(* Logix 5000 AddOnInstructionDefinition export Banner_TL70PS_PD_v6; software revision 33.00 *)

TYPE Banner_TL70PS_Adv_PD_Seg_v6 :   // Advanced process data set for a TL70 Pro Select Segment.
STRUCT
   Animation : SINT;   // 0 = Off, 1 = Steady, 2 = Flash, 3 = Two Color Flash, 4 = Half/Half, 5 = Half/Half Rotate, 6 = Chase, 7 = Intesnity Sweep
   Speed : SINT;   // 0 = Medium, 1 = Slow, 2 = Fast, 3 = Custom
   Pattern : SINT;   // 0 = Normal, 1 = Strobe, 2 = Three Pulse, 3 = SOS, 4 = Random
   Color_1 : SINT;   // 0=Green, 1=Red, 2=Orange, 3=Amber, 4=Yellow, 5=Lime Green, 6=Spring Green, 7=Cyan, 8=Sky Blue, 9=Blue, 10=Violet, 11=Magenta, 12=Rose, 13 = White
   Color_1_Intensity : SINT;   // 0=High, 1=Medium, 2=Low, 3 = Off, 4 = Custom
   Color_2 : SINT;   // 0=Green, 1=Red, 2=Orange, 3=Amber, 4=Yellow, 5=Lime Green, 6=Spring Green, 7=Cyan, 8=Sky Blue, 9=Blue, 10=Violet, 11=Magenta, 12=Rose, 13 = White
   Color_2_Instensity : SINT;   // 0=High, 1=Medium, 2=Low, 3 = Off, 4 = Custom
END_STRUCT
END_TYPE

TYPE Banner_TL70PS_Adv_PDO_v6 :   // Advanced process data set for a TL70 Pro Select IO-Link unit.
STRUCT
   Segment_1 : Banner_TL70PS_Adv_PD_Seg_v6;   // Advanced process data set for a TL70 Segment.
   Segment_2 : Banner_TL70PS_Adv_PD_Seg_v6;   // Advanced process data set for a TL70 Segment.
   Segment_3 : Banner_TL70PS_Adv_PD_Seg_v6;   // Advanced process data set for a TL70 Segment.
   Segment_4 : Banner_TL70PS_Adv_PD_Seg_v6;   // Advanced process data set for a TL70 Segment.
   Segment_5 : Banner_TL70PS_Adv_PD_Seg_v6;   // Advanced process data set for a TL70 Segment.
   Audible_State : SINT;   // 0 = Off, 1 = On
   Audible_Type : SINT;   // 0=Freq, 1=Sync, 2=Off
   Audible_Volume : SINT;   // 0=High, 1=Medium, 2=Low, 3=Off
   Audible_Tone_1 : SINT;   // 0=Freq 3, 1=Freq 2, 2=Freq 1, 3=Off
   Audible_Tone_2 : SINT;   // 0=Freq 3, 1=Freq 2, 2=Freq 1, 3=Off
END_STRUCT
END_TYPE

TYPE Banner_TL70PS_Out_Level_v6 :
STRUCT
   Process_Level : INT;
   Audible_State : SINT;   // 0=Off, 1=On
END_STRUCT
END_TYPE

TYPE Banner_TL70PS_PDO_v6 :   // Process data for a Banner TL70 Pro Select unit. This includes four process data types.
STRUCT
   Segment_PD : Banner_TL70PS_Segment_PD_v6;
   Run_PD : Banner_TL70PS_Run_PD_v6;
   Advanced_PD : Banner_TL70PS_Adv_PDO_v6;
   Out_Level_PD : Banner_TL70PS_Out_Level_v6;
   Transfer_Data : SINT[18];   // Data array to send the correct state of the process data output to the IO-Link master.
END_STRUCT
END_TYPE

TYPE Banner_TL70PS_Run_PD_v6 :   // Run mode process data set for a TL70 Pro Select IO-Link unit.
STRUCT
   Animation : SINT;   // 0 = Off, 1 = Steady, 2 = Flash, 3 = Two Color, 4 = Half/Half, 5 = Half/Half Rotate, 6 = Chase, 7 = Intesnity Sweep, 8 = Scroll, 9 = Bounce, 10 = Demo
   Color_1 : SINT;   // 0 = Green, 1 = Red, 2 = Orange, 3 = Amber, 4 = Yellow, 5 = Lime Green, 6 = Spring Green, 7 = Cyan, 8 = Sky Blue, 9 = Blue, 10 = Violet, 11 = Magenta, 12 = Rose, 13 = White, 14 = Custom, 15 = Custom 2
   Color_1_Intensity : SINT;   // 0 = High, 1 = Low, 2 = Medium, 3 = Off, 4 = Custom
   Speed : SINT;   // 0 = Medium, 1 = Fast, 2 = Slow, 3 = Custom
   Pattern : SINT;   // 0 = Normal, 1 = Strobe, 2 = Three Pulse, 3 = SOS, 4 = Random
   Color_2 : SINT;   // 0 = Green, 1 = Red, 2 = Orange, 3 = Amber, 4 = Yellow, 5 = Lime Green, 6 = Spring Green, 7 = Cyan, 8 = Sky Blue, 9 = Blue, 10 = Violet, 11 = Magenta, 12 = Rose, 13 = White, 14 = Custom, 15 = Custom 2
   Color_2_Intensity : SINT;   // 0 = High, 1 = Low, 2 = Medium, 3 = Off, 4 = Custom
   Direction : SINT;   // 0 = Up, 1 = Down
   Audible : SINT;   // 0 = Off, 1 = On
END_STRUCT
END_TYPE

TYPE Banner_TL70PS_Segment_PD_v6 :   // Basic process data set for a TL70 Pro Select IO-Link unit.
STRUCT
   Segment_1 : SINT;   // 0 = Off, 1 = On, 2 = Flash, 3 = Animation Type
   Segment_2 : SINT;   // 0 = Off, 1 = On, 2 = Flash, 3 = Animation Type
   Segment_3 : SINT;   // 0 = Off, 1 = On, 2 = Flash, 3 = Animation Type
   Segment_4 : SINT;   // 0 = Off, 1 = On, 2 = Flash, 3 = Animation Type
   Segment_5 : SINT;   // 0 = Off, 1 = On, 2 = Flash, 3 = Animation Type
   Audible : SINT;   // 0 = Off, 1 = On
END_STRUCT
END_TYPE

ADD_ON_INSTRUCTION Banner_TL70PS_Adv_PD_v6   (* revision 6.0, vendor Banner Engineering *)
// AOI converts the Advanced process and places it into the correct bytes for transfer to the IO-Link master.
VAR_IN_OUT
   Segment : Banner_TL70PS_Adv_PD_Seg_v6; {required}
   Byte_1 : SINT; {required}
   Byte_2 : SINT; {required}
   Byte_3 : SINT; {required}
END_VAR

ROUTINE Logic   (* ladder *)
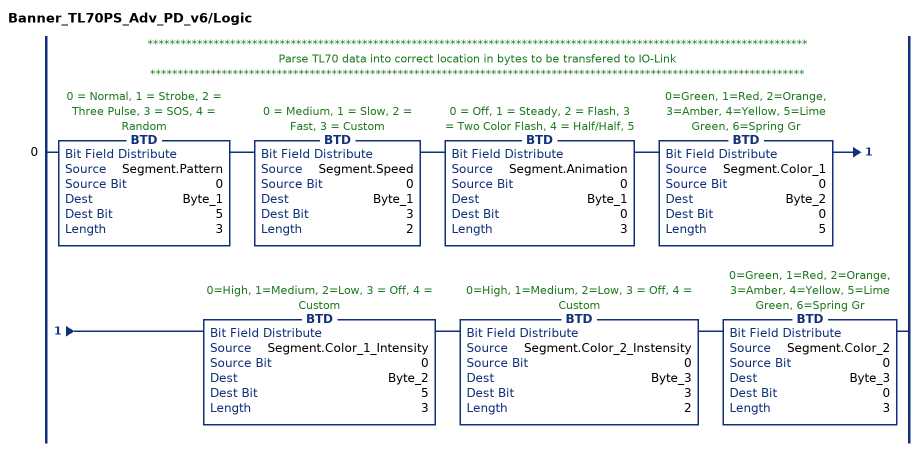
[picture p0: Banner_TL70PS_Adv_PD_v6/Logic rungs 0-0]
   // ************************************************************************************************************************
   // Parse TL70 data into correct location in bytes to be transfered to IO-Link
   // ***********************************************************************************************************************
   0: BTD(Segment.Pattern,0,Byte_1,5,3)BTD(Segment.Speed,0,Byte_1,3,2)BTD(Segment.Animation,0,Byte_1,0,3)BTD(Segment.Color_1,0,Byte_2,0,5)BTD(Segment.Color_1_Intensity,0,Byte_2,5,3)BTD(Segment.Color_2_Instensity,0,Byte_3,3,2)BTD(Segment.Color_2,0,Byte_3,0,3);
END_ROUTINE
END_ADD_ON_INSTRUCTION

ADD_ON_INSTRUCTION Banner_TL70PS_PD_v6   (* revision 6.0, vendor Banner Engineering *)
// Takes the raw SINT information and converts that data into actual information.
VAR_IN_OUT
   PDIO : Banner_TL70PS_PDO_v6; {required}
END_VAR
VAR_INPUT
   Byte_Swap : BOOL; {required}   // Swap the LSB and the MSB with each other.
   Operation_Mode : INT; {required}   // 0 = Segment, 1 = Run, 2 = Level, 3 = Gauge, 4 = Advanced
END_VAR
VAR
   Temp_Measurement : DINT; {access None}
   Data_Byte : SINT[20]; {access None}
   Temp_Data : SINT[20]; {access None}
   AOI_Status : Banner_TL70PS_Adv_PD_v6[10]; {access None}
END_VAR

ROUTINE Logic   (* ladder *)
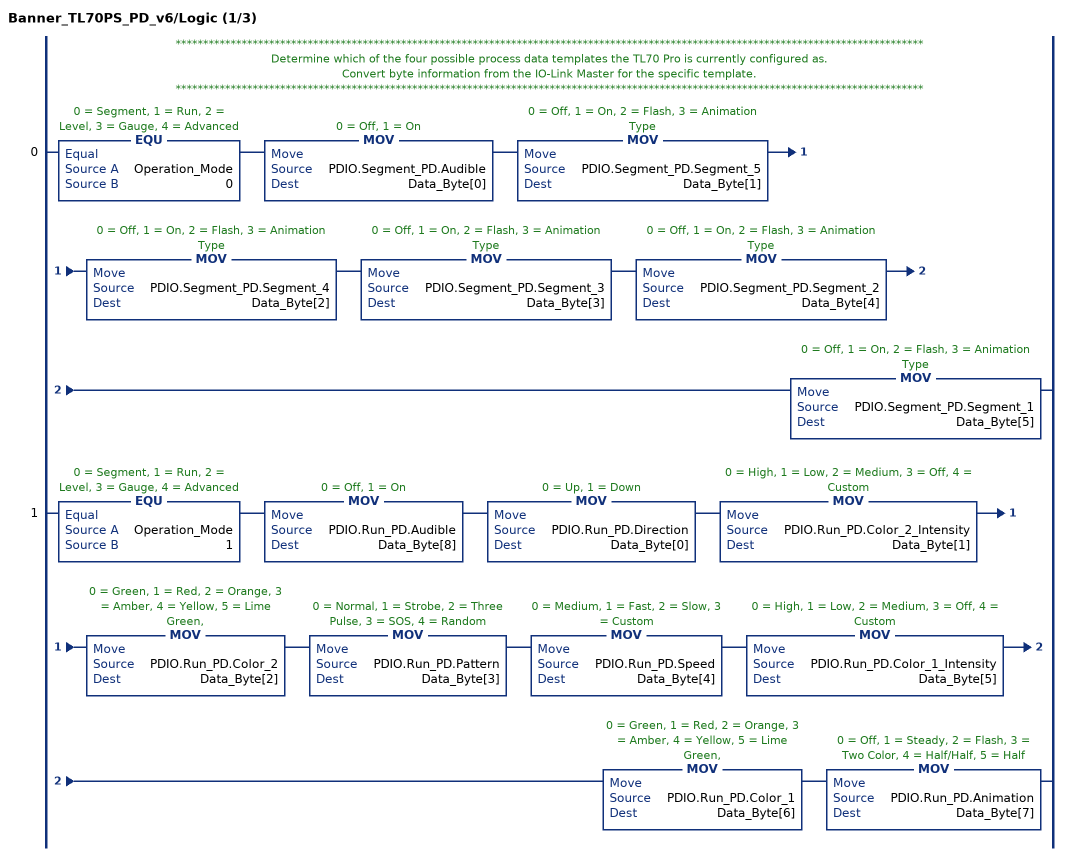
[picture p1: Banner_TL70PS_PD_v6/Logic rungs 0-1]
   // ****************************************************************************************************************************************
   // Determine which of the four possible process data templates the TL70 Pro is currently configured as.
   // Convert byte information from the IO-Link Master for the specific template.
   // ****************************************************************************************************************************************
   0: EQU(Operation_Mode,0)MOV(PDIO.Segment_PD.Audible,Data_Byte[0])MOV(PDIO.Segment_PD.Segment_5,Data_Byte[1])MOV(PDIO.Segment_PD.Segment_4,Data_Byte[2])MOV(PDIO.Segment_PD.Segment_3,Data_Byte[3])MOV(PDIO.Segment_PD.Segment_2,Data_Byte[4])MOV(PDIO.Segment_PD.Segment_1,Data_Byte[5]);
   1: EQU(Operation_Mode,1)MOV(PDIO.Run_PD.Audible,Data_Byte[8])MOV(PDIO.Run_PD.Direction,Data_Byte[0])MOV(PDIO.Run_PD.Color_2_Intensity,Data_Byte[1])MOV(PDIO.Run_PD.Color_2,Data_Byte[2])MOV(PDIO.Run_PD.Pattern,Data_Byte[3])MOV(PDIO.Run_PD.Speed,Data_Byte[4])MOV(PDIO.Run_PD.Color_1_Intensity,Data_Byte[5])MOV(PDIO.Run_PD.Color_1,Data_Byte[6])MOV(PDIO.Run_PD.Animation,Data_Byte[7]);
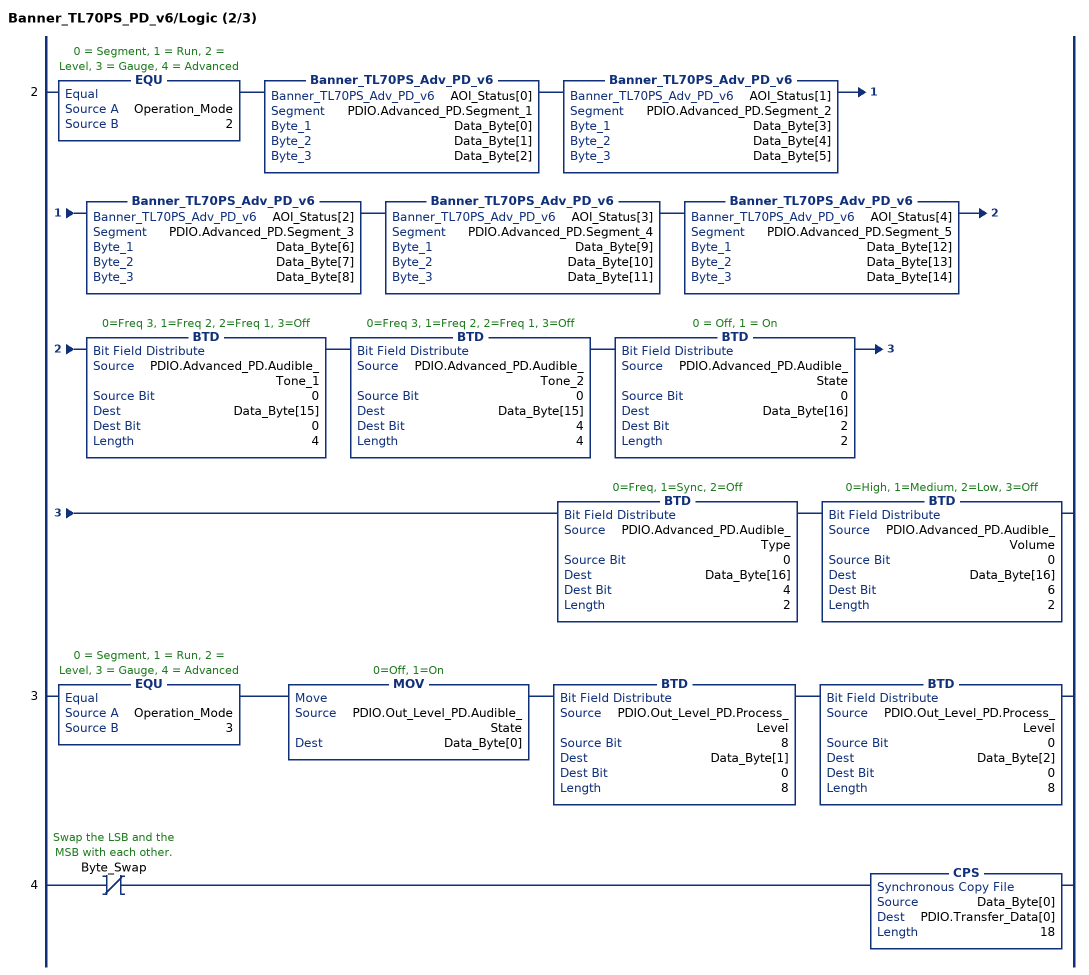
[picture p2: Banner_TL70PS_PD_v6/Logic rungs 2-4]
   2: EQU(Operation_Mode,2)Banner_TL70PS_Adv_PD_v6(AOI_Status[0],PDIO.Advanced_PD.Segment_1,Data_Byte[0],Data_Byte[1],Data_Byte[2])Banner_TL70PS_Adv_PD_v6(AOI_Status[1],PDIO.Advanced_PD.Segment_2,Data_Byte[3],Data_Byte[4],Data_Byte[5])Banner_TL70PS_Adv_PD_v6(AOI_Status[2],PDIO.Advanced_PD.Segment_3,Data_Byte[6],Data_Byte[7],Data_Byte[8])Banner_TL70PS_Adv_PD_v6(AOI_Status[3],PDIO.Advanced_PD.Segment_4,Data_Byte[9],Data_Byte[10],Data_Byte[11])Banner_TL70PS_Adv_PD_v6(AOI_Status[4],PDIO.Advanced_PD.Segment_5,Data_Byte[12],Data_Byte[13],Data_Byte[14])BTD(PDIO.Advanced_PD.Audible_Tone_1,0,Data_Byte[15],0,4)BTD(PDIO.Advanced_PD.Audible_Tone_2,0,Data_Byte[15],4,4)BTD(PDIO.Advanced_PD.Audible_State,0,Data_Byte[16],2,2)BTD(PDIO.Advanced_PD.Audible_Type,0,Data_Byte[16],4,2)BTD(PDIO.Advanced_PD.Audible_Volume,0,Data_Byte[16],6,2);
   3: EQU(Operation_Mode,3)MOV(PDIO.Out_Level_PD.Audible_State,Data_Byte[0])BTD(PDIO.Out_Level_PD.Process_Level,8,Data_Byte[1],0,8)BTD(PDIO.Out_Level_PD.Process_Level,0,Data_Byte[2],0,8);
   4: XIO(Byte_Swap)CPS(Data_Byte[0],PDIO.Transfer_Data[0],18);
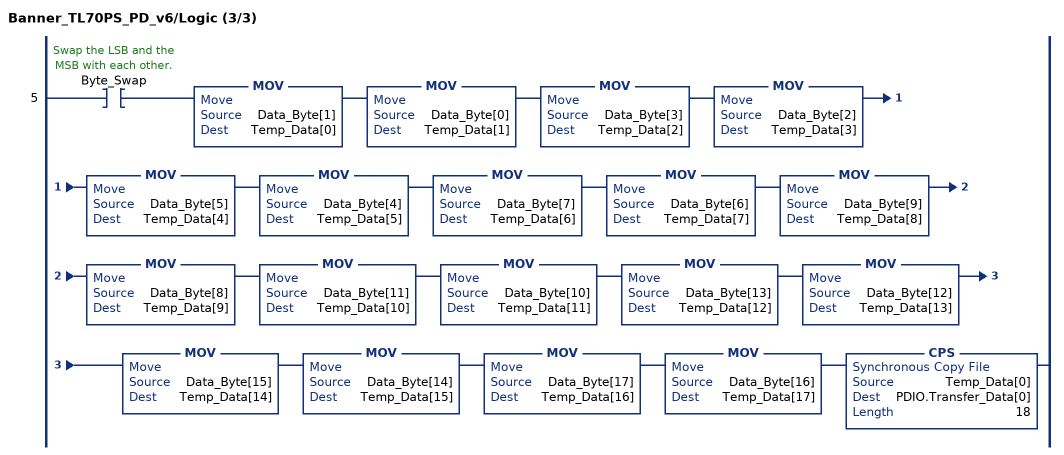
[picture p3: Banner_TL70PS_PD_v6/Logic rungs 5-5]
   5: XIC(Byte_Swap)MOV(Data_Byte[1],Temp_Data[0])MOV(Data_Byte[0],Temp_Data[1])MOV(Data_Byte[3],Temp_Data[2])MOV(Data_Byte[2],Temp_Data[3])MOV(Data_Byte[5],Temp_Data[4])MOV(Data_Byte[4],Temp_Data[5])MOV(Data_Byte[7],Temp_Data[6])MOV(Data_Byte[6],Temp_Data[7])MOV(Data_Byte[9],Temp_Data[8])MOV(Data_Byte[8],Temp_Data[9])MOV(Data_Byte[11],Temp_Data[10])MOV(Data_Byte[10],Temp_Data[11])MOV(Data_Byte[13],Temp_Data[12])MOV(Data_Byte[12],Temp_Data[13])MOV(Data_Byte[15],Temp_Data[14])MOV(Data_Byte[14],Temp_Data[15])MOV(Data_Byte[17],Temp_Data[16])MOV(Data_Byte[16],Temp_Data[17])CPS(Temp_Data[0],PDIO.Transfer_Data[0],18);
END_ROUTINE
END_ADD_ON_INSTRUCTION
